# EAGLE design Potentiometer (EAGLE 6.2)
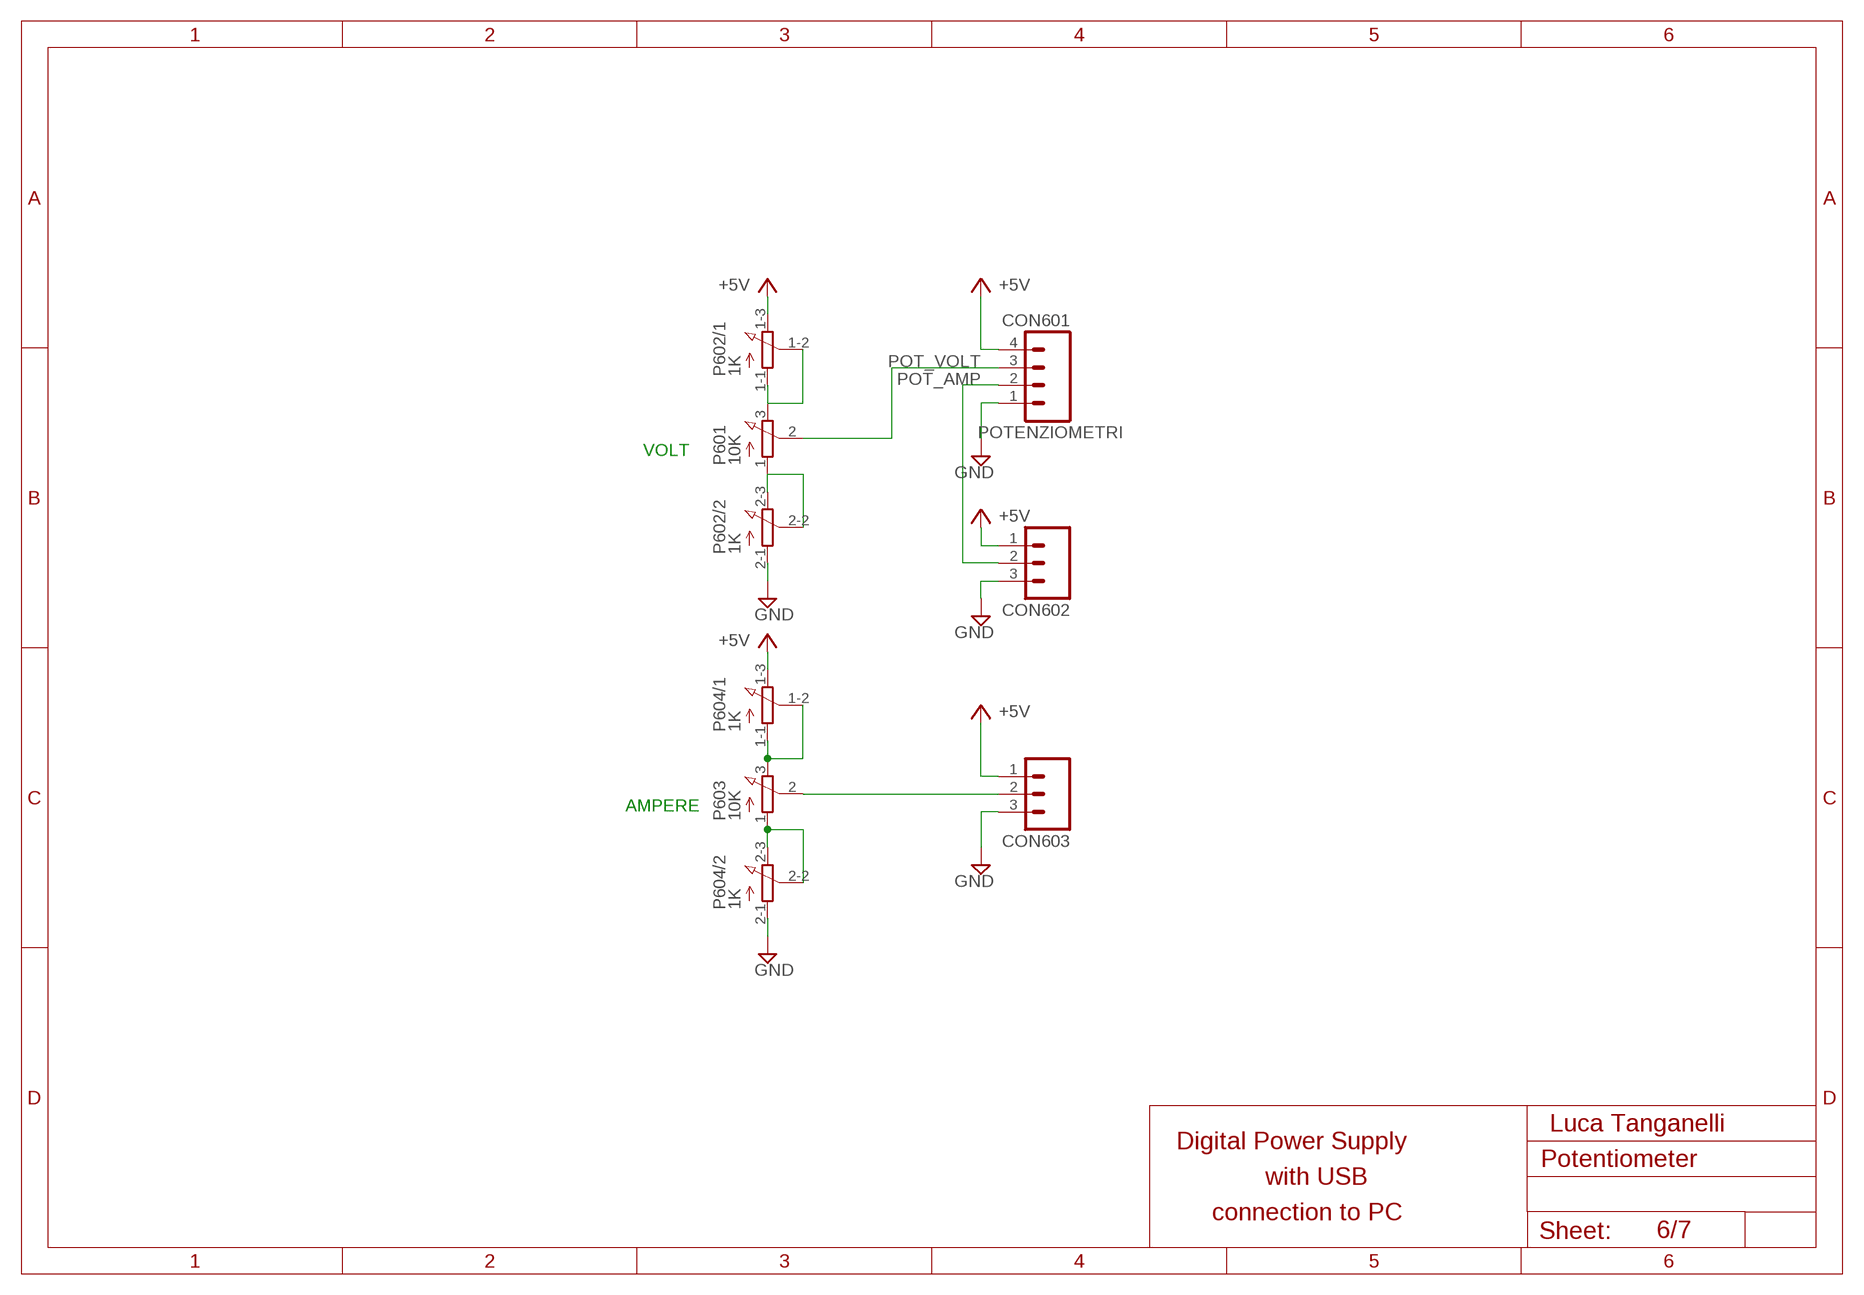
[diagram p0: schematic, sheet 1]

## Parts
CON601  POTENZIOMETRI  M04  [04P]
CON602  M03  [03P]
CON603  M03  [03P]
P601  10K  3RP/1610N  [3RP/1610N]
P602  1K  3RP/1610G  [3RP/1610G]
P603  10K  3RP/1610N  [3RP/1610N]
P604  1K  3RP/1610G  [3RP/1610G]

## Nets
+5V: CON601.4 CON602.1 P602.1-3(/1:E)
+5V_2: CON603.1 P604.1-3(/1:E) ; supply symbol labelled +5V
GND: CON601.1 CON602.3 P602.2-1(/2:A)
GND_2: CON603.3 P604.2-1(/2:A) ; supply symbol labelled GND
N$61: P601.1(A) P602.2-2(/2:S) P602.2-3(/2:E)
N$63: P601.3(E) P602.1-1(/1:A) P602.1-2(/1:S)
N$66: P603.1(A) P604.2-2(/2:S) P604.2-3(/2:E)
N$67: P603.3(E) P604.1-1(/1:A) P604.1-2(/1:S)
N$68: CON603.2 P603.2(S)
POT_AMP: CON601.2 CON602.2
POT_VOLT: CON601.3 P601.2(S)

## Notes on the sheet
- VOLT
- AMPERE
- Luca Tanganelli
- Digital Power Supply
- with USB
- connection to PC
- 6/7

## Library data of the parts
CON601 = #-con-amp-quick:M04: AMP QUICK CONNECTOR; OC_FARNELL: unknown; OC_NEWARK: unknown
CON602 CON603 = #-con-amp-quick:M03: AMP QUICK CONNECTOR; OC_FARNELL: unknown; OC_NEWARK: unknown
P601 P603 = #-pot:3RP/1610N: 16mm Potentiometer one level Source: http://www.alphapotentiometers.net/html/16mm_pot_2.html
P602 P604 = #-pot:3RP/1610G: 16mm Potentiometer two level Source: http://www.alphapotentiometers.net/html/16mm_pot_2.html

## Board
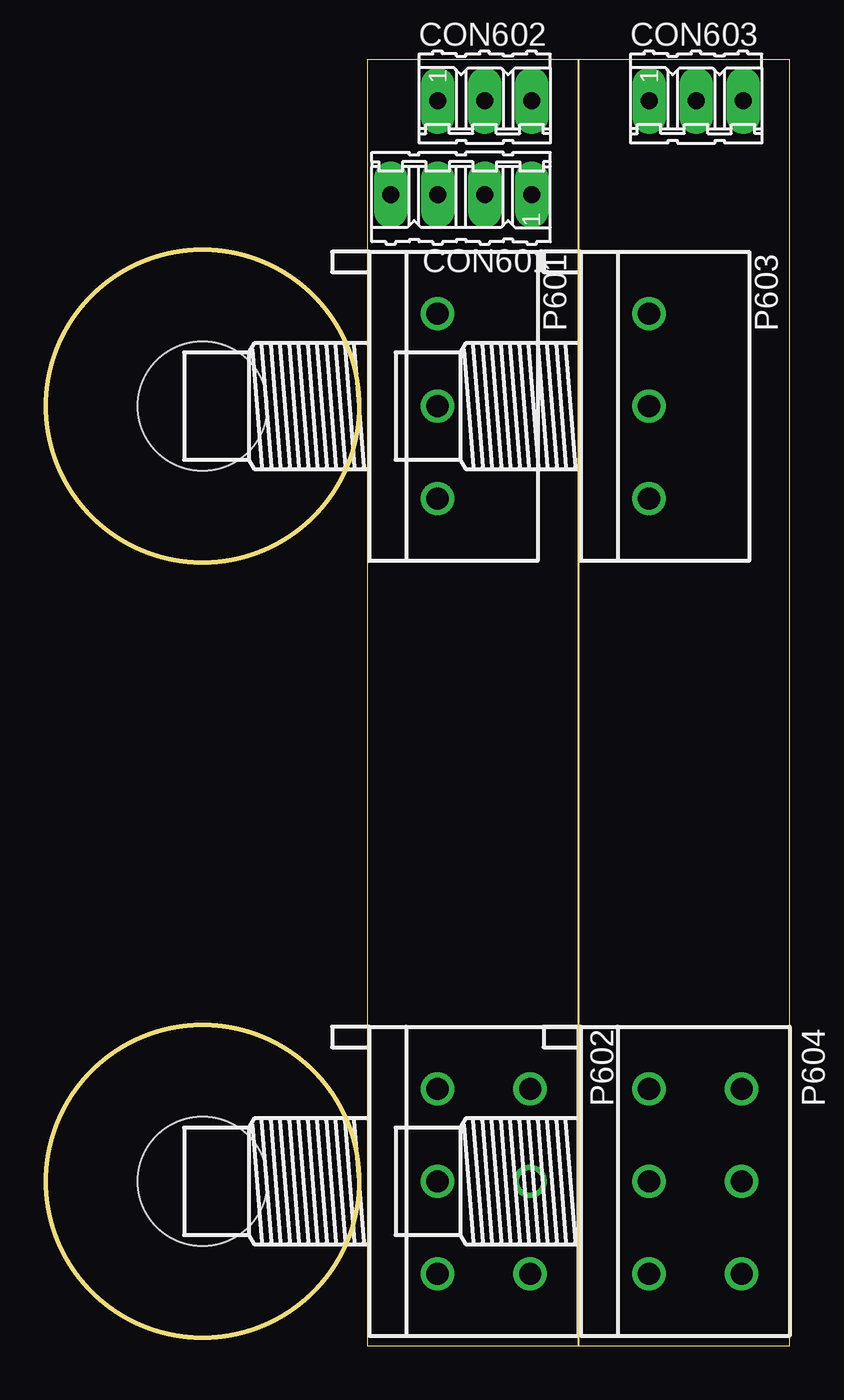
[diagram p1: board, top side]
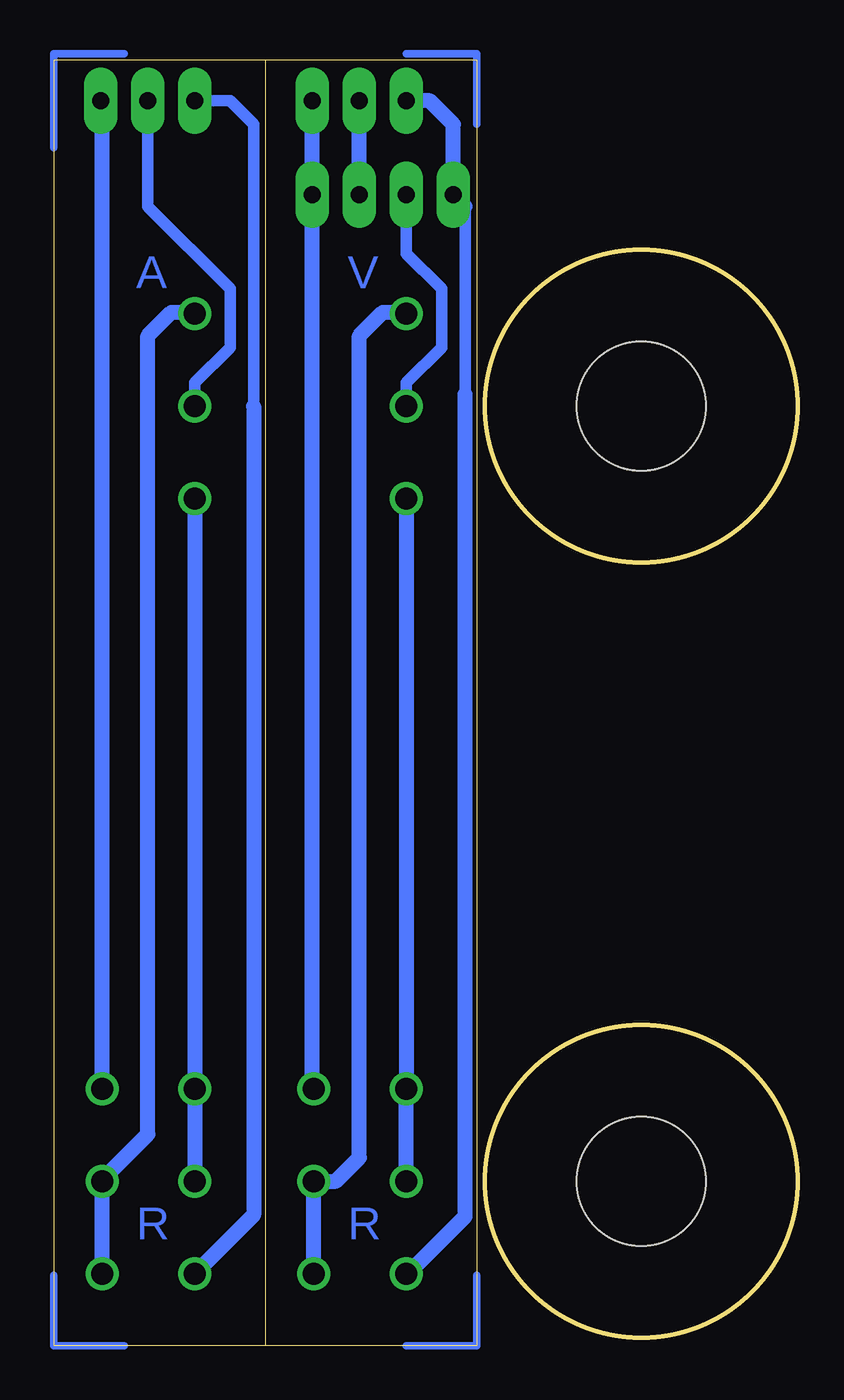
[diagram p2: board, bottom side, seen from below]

Size 40.18 x 69.52 mm. Coordinates in mm from the lower left corner, seen from the top.
Outline: 17.34,0 28.75,0 28.75,69.52 17.34,69.52 17.34,0
Outline: 40.18,0 40.18,69.52 28.77,69.52 28.77,0 40.18,0
Outline: circle at 8.45,50.8 radius 8.45
Outline: circle at 8.45,8.89 radius 8.45
Copper layers (1*16): Top 0.035mm / dielectric 1.5mm / Bottom 0.035mm
Design rules: minimum track width 10mil, minimum drill 24mil, track to track 8mil, track to pad 8mil, pad to pad 8mil, via to via 8mil, smd to smd 8mil, copper to edge 40mil, drill to drill 8mil, minimum pad ring 10mil, minimum via ring 8mil, stop-mask expansion 4mil, vias tented up to drill 0mil, thermal gap 10mil
Holes 7 mm at 8.45,50.8 8.45,8.89

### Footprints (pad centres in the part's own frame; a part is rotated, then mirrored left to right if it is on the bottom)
04P = drill 0.914 pad 1.8 long: 1 -3.81,0; 2 -1.27,0; 3 1.27,0; 4 3.81,0
03P = drill 0.914 pad 1.8 long: 1 -2.54,0; 2 0,0; 3 2.54,0
3RP/1610N = drill 1.2 pad 1.7: 1 -5,0; 2 0,0; 3 5,0
3RP/1610G = drill 1.2 pad 1.7: 1-1 -5,0; 1-2 0,0; 1-3 5,0; 2-1 -5,5; 2-2 0,5; 2-3 5,5

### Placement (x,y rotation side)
CON601  22.42,62.23 180 top
CON602  23.69,67.31 0 top
CON603  35.12,67.31 0 top
P601  21.15,50.8 270 top
P602  21.15,8.89 270 top
P603  32.58,50.8 270 top
P604  32.58,8.89 270 top

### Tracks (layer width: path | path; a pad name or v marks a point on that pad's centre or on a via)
+5V
  Bottom 0.61: 17.98,51.44 17.98,61.59
  Bottom 0.813: P602.1-3 21.07,3.89 17.98,6.99 17.98,51.44 | 17.98,61.59 CON601.4 18.61,66.04 19.88,67.31 CON602.1
+5V_2
  Bottom 0.61: CON603.1 30.68,67.31 29.41,66.04 29.41,50.8
  Bottom 0.813: 29.41,50.8 29.41,7.07 P604.1-3
GND
  Bottom 0.813: P602.2-1 26.23,13.89 CON601.1 CON602.3
GND_2
  Bottom 0.813: P604.2-1 37.58,67.23 CON603.3
N$1
  Bottom 0.406: 17.34,3.81 17.34,0 21.15,0
N$2
  Bottom 0.406: 36.39,0 40.2,0 40.2,3.81
N$3
  Bottom 0.406: 17.34,66.04 17.34,69.85 21.15,69.85
N$4
  Bottom 0.406: 40.2,64.77 40.2,69.85 36.39,69.85
N$61
  Bottom 0.813: P602.2-3 26.15,8.81 26.23,8.89 P602.2-2 24.96,8.89 23.69,10.16 23.69,54.61 22.42,55.88 21.23,55.88 P601.1
N$63
  Bottom 0.813: P601.3 P602.1-1 P602.1-2
N$66
  Bottom 0.813: P604.2-3 P604.2-2 37.58,8.97 35.12,11.43 35.12,54.61 33.85,55.88 32.66,55.88 P603.1
N$67
  Bottom 0.813: P603.3 P604.1-1 P604.1-2
N$68
  Bottom 0.61: CON603.2 35.12,61.59 30.68,57.15 30.68,53.98 32.58,52.07 P603.2
POT_AMP
  Bottom 0.813: CON601.2 CON602.2
POT_VOLT
  Bottom 0.61: P601.2 21.15,52.07 19.25,53.98 19.25,57.15 21.15,59.05 CON601.3

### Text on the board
Bottom: V | A | R | R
